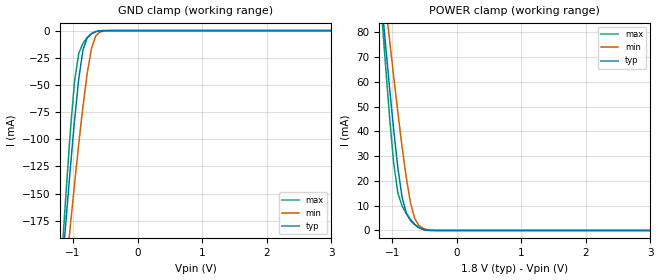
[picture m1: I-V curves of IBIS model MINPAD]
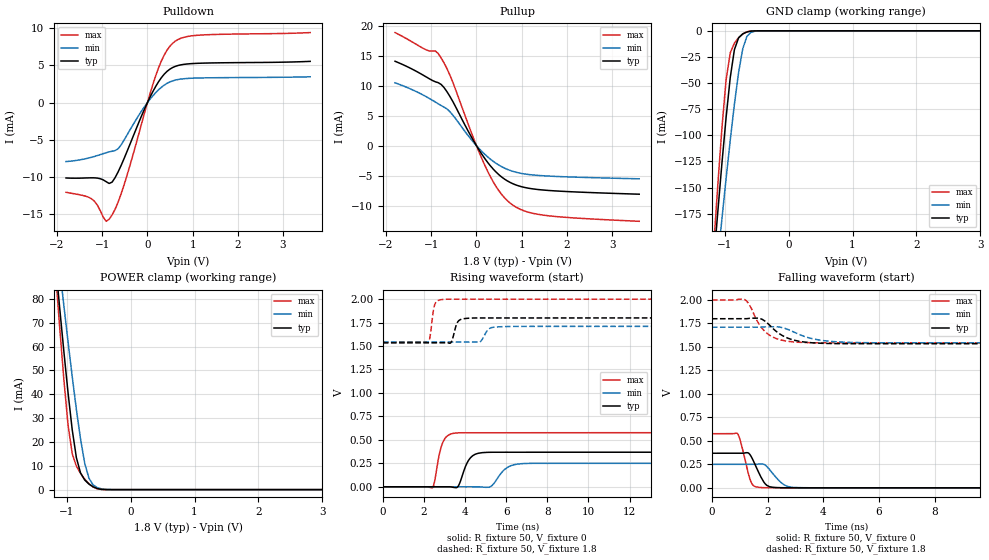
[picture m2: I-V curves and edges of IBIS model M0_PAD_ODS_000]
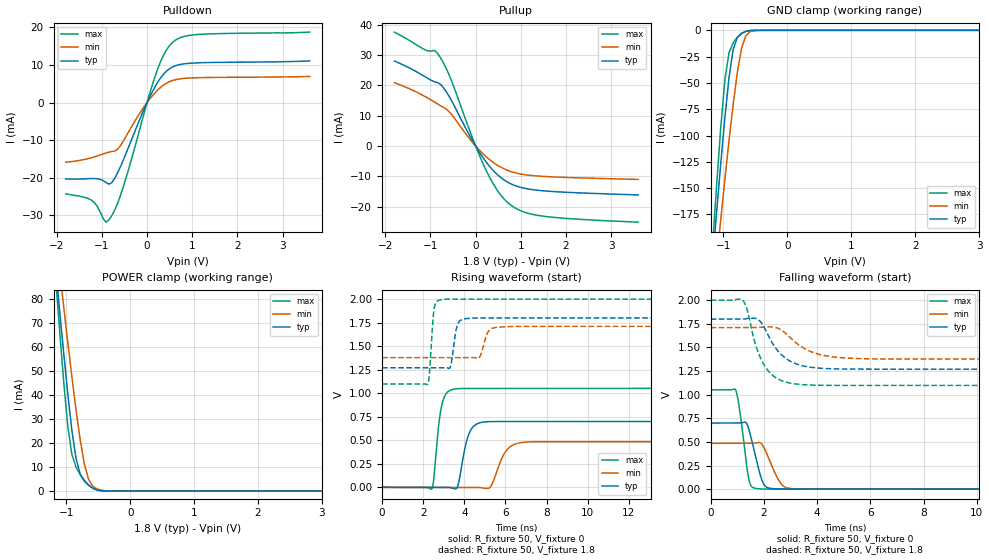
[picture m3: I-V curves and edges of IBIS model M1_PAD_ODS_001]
| Created by SiliconSmart  S-2021.06-SP5-2
[IBIS Ver]   4.0
[File Name]   as320ck_18v_rev1p2.ibs
[File Rev]   1.2
[Date]   Wed Apr 02 2025
|[Source]   Avalanche Team
|[Notes]   Generated IBIS models from Silicon Smart
|[Rev 1.0]   Initial release based on extracted netlist
|[Rev 1.1]   Updated the VCC supply values according to
|		datasheet
|[Rev 1.2]   Updated the ODS models
|[Disclaimer]   THE MODEL LIBRARIES ARE PROVIDED AS IS.
|[Copyright]   Copyright 2024, Avalanche Technology, All Rights Reserved
[Component]   AS30XX20X_BGA
[Manufacturer]  Avalanche Technology
| CONTENT :
| This file contains IBIS MODEL for PSRAM device
| AS30XX20X
| USAGE :
| The models are derived for the 1.71V to 2.0V I/O Operation.
| Temperatures for model generation: typ: 25, max: -40, min: 125
| Voltages : typ: 1.8V, min: 1.71V, max: 2.0V
| PACKAGES SUPPORTED :
| 56-ball FBGA (10mm x 10mm)
| VERIFICATION
| Errors  : 0
| Warnings: 19
| All warnings due to non-monotonic data:
[Package]
|  Design die-package: BGA
| variable   typ   min   max
R_pkg   0.72029   0.51528   1.0002
L_pkg   5.797e-9   4.155e-9   8.073e-9
C_pkg   1.116e-12   7.907e-13   1.753e-12
|Pin and Model info
[Pin]  signal_name  model_name   R_pin   L_pin   C_pin
E2   CS1#   MINPAD   0.4340	15.2000E-9	1.2600E-12
C3   CS2#   MINPAD   0.3800	13.5000E-9	1.0400E-12
D2   CLK1   MINPAD   0.4300	12.7000E-9	0.9790E-12
D1   CLK2   MINPAD   0.4480	14.6000E-9	1.1600E-12
F3   IO_0   MIOPAD   0.4010	12.4000E-9	1.2500E-12
F2   IO_1   MIOPAD   0.4050	14.2000E-9	1.1100E-12
E4   IO_2   MIOPAD   0.3780	11.8000E-9	1.2000E-12
F4   IO_3   MIOPAD   0.3700	11.8000E-9	1.2600E-12
F5   IO_4   MIOPAD   0.3710	11.1000E-9	1.1000E-12
G3   IO_5   MIOPAD   0.4050	13.8000E-9	1.1600E-12
G2   IO_6   MIOPAD   0.3830	15.2000E-9	1.0900E-12
G1   IO_7   MIOPAD   0.4480	16.4000E-9	1.0800E-12
C7   HTBSEL   MINPAD   0.1380	6.1700E-9	0.6060E-12
B7   HBP_2   MINPAD   0.1470	6.3900E-9	1.0000E-12
A6   HBP_1   MINPAD   0.1910	8.5000E-9	1.1500E-12
A5   HBP_0   MINPAD   0.2050	8.6800E-9	1.4200E-12
C4   RESET#   MINPAD   0.3410	14.1000E-9	1.6300E-12
C5   INT1#   MIOPAD   0.3080	12.5000E-9	1.2100E-12
D3   INT2#   MIOPAD   0.2120	10.3000E-9	0.8230E-12
B1   VSSIO   GND   NA   NA   NA
B5   VSSIO   GND   NA   NA   NA
B6   VSSIO   GND   NA   NA   NA
E1   VSSIO   GND   NA   NA   NA
G5   VSSIO   GND   NA   NA   NA
G6   VSSIO   GND   NA   NA   NA
A1   VSS   GND   NA   NA   NA
A3   VSS   GND   NA   NA   NA
B3   VSS   GND   NA   NA   NA
E5   VSS   GND   NA   NA   NA
E6   VSS   GND   NA   NA   NA
E7   VSS   GND   NA   NA   NA
G7   VSS   GND   NA   NA   NA
A8   VSS   GND   NA   NA   NA
A7   VCCIO   POWER   NA   NA   NA
B2   VCCIO   POWER   NA   NA   NA
B4   VCCIO   POWER   NA   NA   NA
C6   VCCIO   POWER   NA   NA   NA
F1   VCCIO   POWER   NA   NA   NA
F6   VCCIO   POWER   NA   NA   NA
G4   VCCIO   POWER   NA   NA   NA
A2   VCC   POWER   NA   NA   NA
A4   VCC   POWER   NA   NA   NA
D4   VCC   POWER   NA   NA   NA
D6   VCC   POWER   NA   NA   NA
D7   VCC   POWER   NA   NA   NA
F7   VCC   POWER   NA   NA   NA
| IOPAD
[Model Selector] MIOPAD
| Model Description
M0_PAD_ODS_000   ODS_000
M1_PAD_ODS_001   ODS_001
M2_PAD_ODS_010   ODS_010
M3_PAD_ODS_011   ODS_011
M4_PAD_ODS_100   ODS_100
M5_PAD_ODS_101   ODS_101
M6_PAD_ODS_110   ODS_110
M7_PAD_ODS_111   ODS_111
| Models and submodels in the file (9): MINPAD (Input), M0_PAD_ODS_000 (I/O), M1_PAD_ODS_001 (I/O), M2_PAD_ODS_010 (I/O), M3_PAD_ODS_011 (I/O), M4_PAD_ODS_100 (I/O), M5_PAD_ODS_101 (I/O), M6_PAD_ODS_110 (I/O), M7_PAD_ODS_111 (I/O)
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[Model] MINPAD
Model_type Input
Enable   Active-High
Vinl  =  0.63
Vinh  =  1.17
| Capacitance  typ   min   max
C_comp   1.623824e-12   1.523246e-12   1.739467e-12
| Variables   typ   min   max
[GND Clamp Reference]   0   0   0
[POWER Clamp Reference]   1.8   1.71   2
[Pulldown Reference]   0   0   0
[Pullup Reference]   1.8   1.71   2
[Temperature Range]   25   125   -40
[Voltage Range]   1.8   1.71   2
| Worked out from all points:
|   GND clamp passes 1 mA (typ) near -0.64 V on its own axis
|   POWER clamp passes 1 mA (typ) near -0.57 V on its own axis
[GND Clamp]
| Voltage   I(typ)   I(min)   I(max)
-1.8V     -720.4mA   -670.5mA   -825.2mA
-1.173V   -222.3mA   -260.3mA   -207.5mA
-1.108V   -173.8mA   -219.8mA   -148.3mA
-1.043V   -126.9mA   -180.1mA   -93.11mA
-977.6mV  -83.02mA   -141.5mA   -47mA
-912.4mV  -44.68mA   -104.6mA   -21.04mA
-847.2mV  -17.95mA   -70.1mA    -11.75mA
-782.1mV  -6.736mA   -39.85mA   -6.524mA
-716.9mV  -2.917mA   -17.13mA   -2.959mA
-651.7mV  -1.107mA   -5.246mA   -906.9uA
-456.2mV  -3.885uA   -74.14uA   -372.9nA
3.6V      0A         0A         0A
[POWER Clamp]
| Voltage   I(typ)   I(min)   I(max)
-1.8V     287.1mA    268.3mA    329.6mA
-1.173V   94.89mA    108.5mA    91.02mA
-1.108V   76.1mA     92.66mA    67.97mA
-1.043V   57.9mA     77.16mA    46.14mA
-977.6mV  40.62mA    62.05mA    27.14mA
-912.4mV  25.13mA    47.46mA    15.06mA
-847.2mV  13.38mA    33.64mA    9.853mA
-716.9mV  4.014mA    11.09mA    4.394mA
-651.7mV  2.34mA     4.821mA    2.483mA
-586.6mV  1.18mA     2.003mA    1.113mA
-325.9mV  1.153uA    19.85uA    110.1nA
3.6V      0A         0A         0A
[Model] M0_PAD_ODS_000
Model_type I/O
Enable   Active-High
Vinl  =  0.63
Vinh  =  1.17
Vmeas =  0.9
Cref  =  30e-12
| Capacitance  typ   min   max
C_comp   1.624629e-12   1.520611e-12   1.744819e-12
| Variables   typ   min   max
[GND Clamp Reference]   0   0   0
[POWER Clamp Reference]   1.8   1.71   2
[Pulldown Reference]   0   0   0
[Pullup Reference]   1.8   1.71   2
[Temperature Range]   25   125   -40
[Voltage Range]   1.8   1.71   2
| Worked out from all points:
|   slope of the pulldown table from 0 to 0.27 V, typ, clamps not added: 89.8 ohm
|   slope of the pullup table from 0 to 0.27 V, typ, clamps not added: 90.2 ohm
|   GND clamp passes 1 mA (typ) near -0.64 V on its own axis
|   POWER clamp passes 1 mA (typ) near -0.57 V on its own axis
|   falling waveform, R_fixture 50, V_fixture 0: 20-80 % time 364ps typ, 457ps min, 286ps max; typ from 0.368 V to 0 V
|   falling waveform, R_fixture 50, V_fixture 1.8: 20-80 % time 772ps typ, 993ps min, 609ps max; typ from 1.8 V to 1.53 V
|   rising waveform, R_fixture 50, V_fixture 0: 20-80 % time 416ps typ, 571ps min, 331ps max; typ from 0 V to 0.368 V
|   rising waveform, R_fixture 50, V_fixture 1.8: 20-80 % time 214ps typ, 282ps min, 164ps max; typ from 1.53 V to 1.8 V
[GND Clamp]
| Voltage   I(typ)   I(min)   I(max)
-1.8V     -720.4mA   -670.5mA   -825.2mA
-1.173V   -222.3mA   -260.3mA   -207.5mA
-1.108V   -173.8mA   -219.8mA   -148.3mA
-1.043V   -126.9mA   -180.1mA   -93.11mA
-977.6mV  -83.02mA   -141.5mA   -47.01mA
-912.4mV  -44.68mA   -104.6mA   -21.04mA
-847.2mV  -17.95mA   -70.1mA    -11.75mA
-782.1mV  -6.736mA   -39.85mA   -6.526mA
-716.9mV  -2.917mA   -17.13mA   -2.96mA
-651.7mV  -1.107mA   -5.246mA   -907.6uA
-456.2mV  -3.886uA   -74.14uA   -373.5nA
3.6V      0A         0A         0A
[POWER Clamp]
| Voltage   I(typ)   I(min)   I(max)
-1.8V     287.1mA    268.3mA    329.6mA
-1.173V   94.89mA    108.5mA    91.02mA
-1.108V   76.1mA     92.66mA    67.97mA
-1.043V   57.9mA     77.16mA    46.14mA
-977.6mV  40.62mA    62.05mA    27.14mA
-912.4mV  25.13mA    47.46mA    15.06mA
-847.2mV  13.38mA    33.64mA    9.853mA
-716.9mV  4.014mA    11.09mA    4.394mA
-651.7mV  2.34mA     4.821mA    2.483mA
-586.6mV  1.18mA     2.003mA    1.113mA
-325.9mV  1.153uA    19.85uA    110.1nA
3.6V      0A         0A         0A
[Pulldown]
| Voltage   I(typ)   I(min)   I(max)
-1.8V     -10.11mA   -7.903mA   -12.02mA
-1.238V   -10.08mA   -7.332mA   -12.89mA
-912.4mV  -10.6mA    -6.719mA   -15.91mA
-847.2mV  -10.84mA   -6.607mA   -15.64mA
-716.9mV  -10.08mA   -6.433mA   -14.32mA
-521.4mV  -7.576mA   -5.077mA   -11.12mA
-65.17mV  -872uA     -545.4uA   -1.404mA
248.3mV   2.817mA    1.73mA     4.683mA
434.5mV   4.193mA    2.586mA    7.041mA
620.7mV   4.869mA    3.026mA    8.258mA
1.179V    5.284mA    3.307mA    9.058mA
3.6V      5.531mA    3.462mA    9.391mA
[Pullup]
| Voltage   I(typ)   I(min)   I(max)
-1.8V     14.09mA    10.49mA    18.88mA
-1.108V   11.46mA    8.165mA    15.99mA
-912.4mV  10.68mA    7.305mA    15.83mA
-782.1mV  10.23mA    6.709mA    14.67mA
-586.6mV  8.225mA    5.675mA    11.78mA
-65.17mV  837.2uA    571.9uA    1.256mA
248.3mV   -2.788mA   -1.868mA   -4.273mA
496.6mV   -4.844mA   -3.246mA   -7.521mA
744.8mV   -6.13mA    -4.13mA    -9.572mA
1.055V    -6.951mA   -4.705mA   -10.87mA
1.49V     -7.407mA   -5.024mA   -11.6mA
3.6V      -8.097mA   -5.528mA   -12.62mA
[Ramp]
dV/dt_r   0.221023/0.415541n  0.150294/0.570736n  0.34588/0.331259n
dV/dt_f   0.159898/0.772458n  0.100157/0.992769n  0.274317/0.608956n
R_load = 50
[Falling Waveform]
R_fixture = 50
V_fixture = 0
V_fixture_min = 0
V_fixture_max = 0
| Time   V(typ)   V(min)   V(max)
0s        368.4mV    250.5mV    576.5mV
917.7ps   368.8mV    250.7mV    577.9mV
1.025ns   368.8mV    250.8mV    496.9mV
1.4ns     338.8mV    250.9mV    66.57mV
1.498ns   281.8mV    250.9mV    22.51mV
1.747ns   123.1mV    255.1mV    3.988mV
2.065ns   13.03mV    196.9mV    1.112mV
2.606ns   1.316mV    29.83mV    229.5uV
3.024ns   433.5uV    3.545mV    224.5uV
21.88ns   79.75nV    25.29nV    -226nV
[Falling Waveform]
R_fixture = 50
V_fixture = 1.8
V_fixture_min = 1.71
V_fixture_max = 2
| Time   V(typ)   V(min)   V(max)
0s        1.8V       1.71V      2V
1.175ns   1.8V       1.71V      2.005V
1.306ns   1.803V     1.71V      1.967V
1.72ns    1.803V     1.711V     1.731V
1.981ns   1.756V     1.714V     1.644V
2.418ns   1.642V     1.711V     1.579V
2.948ns   1.572V     1.658V     1.552V
3.916ns   1.539V     1.571V     1.544V
5.337ns   1.534V     1.546V     1.543V
21.88ns   1.534V     1.543V     1.543V
[Rising Waveform]
R_fixture = 50
V_fixture = 0
V_fixture_min = 0
V_fixture_max = 0
| Time   V(typ)   V(min)   V(max)
0s        2.923nV    85.23nV    2.501nV
2.41ns    -265.6uV   -270.7uV   -11.22mV
2.91ns    -320.8uV   -327uV     469.9mV
3.456ns   -7.235mV   -388.3uV   570.2mV
3.683ns   11.84mV    -413.8uV   574.5mV
4.261ns   309.1mV    -478.8uV   575.7mV
4.837ns   363.6mV    -3.076mV   575.7mV
6.059ns   367.9mV    206.6mV    575.8mV
6.73ns    367.9mV    245.7mV    575.8mV
21.88ns   368.4mV    250.5mV    576.5mV
[Rising Waveform]
R_fixture = 50
V_fixture = 1.8
V_fixture_min = 1.71
V_fixture_max = 2
| Time   V(typ)   V(min)   V(max)
0s        1.534V     1.543V     1.543V
2.209ns   1.534V     1.543V     1.54V
2.511ns   1.534V     1.543V     1.934V
2.877ns   1.534V     1.543V     1.996V
3.303ns   1.535V     1.543V     2V
3.663ns   1.763V     1.543V     2V
4.153ns   1.796V     1.542V     2V
4.701ns   1.799V     1.542V     2V
5.68ns    1.799V     1.705V     2V
21.88ns   1.8V       1.71V      2V
[Model] M1_PAD_ODS_001
Model_type I/O
Enable   Active-High
Vinl  =  0.63
Vinh  =  1.17
Vmeas =  0.9
Cref  =  30e-12
| Capacitance  typ   min   max
C_comp   1.624629e-12   1.520611e-12   1.744819e-12
| Variables   typ   min   max
[GND Clamp Reference]   0   0   0
[POWER Clamp Reference]   1.8   1.71   2
[Pulldown Reference]   0   0   0
[Pullup Reference]   1.8   1.71   2
[Temperature Range]   25   125   -40
[Voltage Range]   1.8   1.71   2
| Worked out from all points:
|   slope of the pulldown table from 0 to 0.27 V, typ, clamps not added: 44.9 ohm
|   slope of the pullup table from 0 to 0.27 V, typ, clamps not added: 45.3 ohm
|   GND clamp passes 1 mA (typ) near -0.64 V on its own axis
|   POWER clamp passes 1 mA (typ) near -0.57 V on its own axis
|   falling waveform, R_fixture 50, V_fixture 0: 20-80 % time 369ps typ, 461ps min, 285ps max; typ from 0.7 V to 0 V
|   falling waveform, R_fixture 50, V_fixture 1.8: 20-80 % time 819ps typ, 1.04ns min, 647ps max; typ from 1.8 V to 1.27 V
|   rising waveform, R_fixture 50, V_fixture 0: 20-80 % time 407ps typ, 569ps min, 308ps max; typ from 0 V to 0.7 V
|   rising waveform, R_fixture 50, V_fixture 1.8: 20-80 % time 214ps typ, 282ps min, 165ps max; typ from 1.27 V to 1.8 V
[GND Clamp]
| Voltage   I(typ)   I(min)   I(max)
-1.8V     -720.4mA   -670.5mA   -825.2mA
-1.173V   -222.3mA   -260.3mA   -207.5mA
-1.108V   -173.8mA   -219.8mA   -148.3mA
-1.043V   -126.9mA   -180.1mA   -93.11mA
-977.6mV  -83.02mA   -141.5mA   -47.01mA
-912.4mV  -44.68mA   -104.6mA   -21.04mA
-847.2mV  -17.95mA   -70.1mA    -11.75mA
-782.1mV  -6.736mA   -39.85mA   -6.526mA
-716.9mV  -2.917mA   -17.13mA   -2.96mA
-651.7mV  -1.107mA   -5.246mA   -907.6uA
-456.2mV  -3.886uA   -74.14uA   -373.5nA
3.6V      0A         0A         0A
[POWER Clamp]
| Voltage   I(typ)   I(min)   I(max)
-1.8V     287.1mA    268.3mA    329.6mA
-1.173V   94.89mA    108.5mA    91.02mA
-1.108V   76.1mA     92.66mA    67.97mA
-1.043V   57.9mA     77.16mA    46.14mA
-977.6mV  40.62mA    62.05mA    27.14mA
-912.4mV  25.13mA    47.46mA    15.06mA
-847.2mV  13.38mA    33.64mA    9.853mA
-716.9mV  4.014mA    11.09mA    4.394mA
-651.7mV  2.34mA     4.821mA    2.483mA
-586.6mV  1.18mA     2.003mA    1.113mA
-325.9mV  1.153uA    19.85uA    110.1nA
3.6V      0A         0A         0A
[Pulldown]
| Voltage   I(typ)   I(min)   I(max)
-1.8V     -20.29mA   -15.84mA   -24.25mA
-1.238V   -20.19mA   -14.67mA   -25.87mA
-912.4mV  -21.19mA   -13.43mA   -31.79mA
-847.2mV  -21.68mA   -13.2mA    -31.24mA
-716.9mV  -20.15mA   -12.86mA   -28.61mA
-521.4mV  -15.14mA   -10.15mA   -22.2mA
-65.17mV  -1.742mA   -1.091mA   -2.802mA
248.3mV   5.63mA     3.46mA     9.353mA
434.5mV   8.383mA    5.171mA    14.07mA
620.7mV   9.735mA    6.051mA    16.51mA
1.179V    10.57mA    6.614mA    18.12mA
3.6V      11.06mA    6.923mA    18.71mA
[Pullup]
| Voltage   I(typ)   I(min)   I(max)
-1.8V     28.07mA    20.9mA     37.6mA
-1.108V   22.77mA    16.25mA    31.67mA
-912.4mV  21.23mA    14.53mA    31.58mA
-782.1mV  20.42mA    13.35mA    29.27mA
-586.6mV  16.4mA     11.32mA    23.49mA
-65.17mV  1.669mA    1.14mA     2.505mA
248.3mV   -5.556mA   -3.722mA   -8.519mA
496.6mV   -9.653mA   -6.467mA   -14.99mA
744.8mV   -12.21mA   -8.229mA   -19.08mA
1.055V    -13.85mA   -9.372mA   -21.68mA
1.49V     -14.76mA   -10.01mA   -23.13mA
3.6V      -16.13mA   -11mA      -25.12mA
[Ramp]
dV/dt_r   0.419845/0.40709n  0.290904/0.569117n  0.630672/0.308383n
dV/dt_f   0.317972/0.818691n  0.199636/1.04487n  0.541445/0.646878n
R_load = 50
[Falling Waveform]
R_fixture = 50
V_fixture = 0
V_fixture_min = 0
V_fixture_max = 0
| Time   V(typ)   V(min)   V(max)
0s        699.7mV    484.8mV    1.051V
936.6ps   700.2mV    485.3mV    1.051V
1.089ns   700.3mV    485.4mV    839.3mV
1.43ns    639mV      485.6mV    108.6mV
1.732ns   294.8mV    491.4mV    6.152mV
1.952ns   76.13mV    465.2mV    2.032mV
2.096ns   21.34mV    384.1mV    1.262mV
2.616ns   1.831mV    69mV       474.1uV
3.058ns   724uV      5.937mV    463.2uV
21.88ns   1.404nV    117.1nV    -317.4nV
[Falling Waveform]
R_fixture = 50
V_fixture = 1.8
V_fixture_min = 1.71
V_fixture_max = 2
| Time   V(typ)   V(min)   V(max)
0s        1.8V       1.71V      2V
1.173ns   1.801V     1.71V      2.008V
1.362ns   1.807V     1.711V     1.909V
1.709ns   1.807V     1.711V     1.511V
2.045ns   1.695V     1.717V     1.297V
2.543ns   1.458V     1.701V     1.165V
3.19ns    1.329V     1.553V     1.114V
4.145ns   1.28V      1.423V     1.1V
5.594ns   1.271V     1.382V     1.098V
21.88ns   1.27V      1.377V     1.098V
[Rising Waveform]
R_fixture = 50
V_fixture = 0
V_fixture_min = 0
V_fixture_max = 0
| Time   V(typ)   V(min)   V(max)
0s        2.363nV    66.36nV    1.939nV
2.414ns   -364.9uV   -508uV     -18.9mV
2.899ns   -438.2uV   -609.9uV   867.9mV
3.517ns   -14.89mV   -740.1uV   1.045V
3.717ns   42.31mV    -782.1uV   1.049V
4.27ns    590.4mV    -898.5uV   1.05V
4.904ns   692.4mV    -7.095mV   1.05V
6.058ns   699mV      394.8mV    1.05V
6.727ns   699mV      474.1mV    1.05V
21.88ns   699.7mV    484.8mV    1.051V
[Rising Waveform]
R_fixture = 50
V_fixture = 1.8
V_fixture_min = 1.71
V_fixture_max = 2
| Time   V(typ)   V(min)   V(max)
0s        1.27V      1.377V     1.098V
2.212ns   1.271V     1.378V     1.092V
2.54ns    1.271V     1.378V     1.907V
2.88ns    1.271V     1.378V     1.994V
3.308ns   1.272V     1.378V     1.999V
3.649ns   1.714V     1.378V     1.999V
4.093ns   1.793V     1.378V     1.999V
4.72ns    1.799V     1.377V     1.999V
5.677ns   1.799V     1.701V     1.999V
21.88ns   1.8V       1.71V      2V
